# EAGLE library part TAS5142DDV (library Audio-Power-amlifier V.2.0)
STEREO DIGITAL AMPLIFIER POWER STAGE
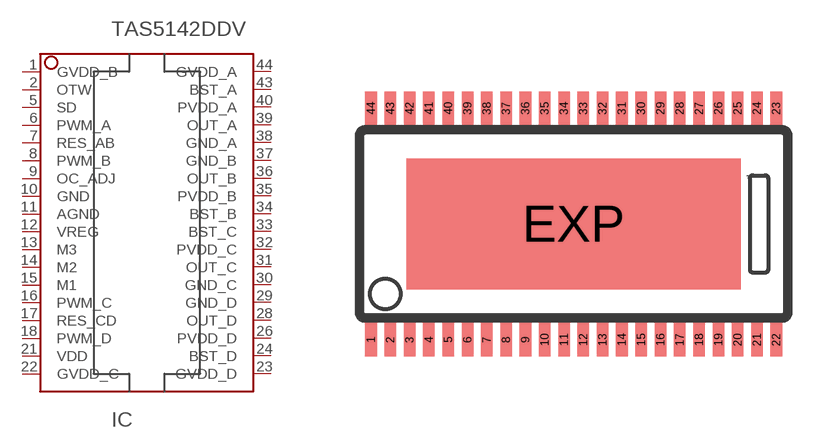
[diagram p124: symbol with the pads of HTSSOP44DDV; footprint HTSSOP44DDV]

Designator prefix IC

## TAS5142DDV  [HTSSOP44DDV]
1  GVDD_B
2  OTW  out
5  SD  out
6  PWM_A  in
7  RES_AB  in
8  PWM_B  in
9  OC_ADJ  out
10  GND  pwr
11  AGND  pwr
12  VREG  pwr
13  M3  in
14  M2  in
15  M1  in
16  PWM_C  in
17  RES_CD  in
18  PWM_D  in
21  VDD  pwr
22  GVDD_C  pwr
23  GVDD_D  pwr
24  BST_D  pwr
26  PVDD_D  pwr
28  OUT_D  out
29  GND_D  pwr
30  GND_C  pwr
31  OUT_C  out
32  PVDD_C  pwr
33  BST_C  pwr
34  BST_B  pwr
35  PVDD_B  pwr
36  OUT_B  out
37  GND_B  pwr
38  GND_A  pwr
39  OUT_A  out
40  PVDD_A  pwr
43  BST_A  pwr
44  GVDD_A  pwr

## Footprint HTSSOP44DDV (pad centres in mm)
PowerPAD(TM) PLASTIC SMALL-OUTLINE PACKAGE DDV (R-PDSO-G**) Source: http://focus.ti.com/lit/ml/mpds041b/mpds041b.pdf / slma002.pdf
smd 0.38 x 1.1: 1 -6.668,-3.81; 2 -6.032,-3.81; 3 -5.397,-3.81; 4 -4.763,-3.81; 5 -4.128,-3.81; 6 -3.493,-3.81; 7 -2.857,-3.81; 8 -2.223,-3.81; 9 -1.587,-3.81; 10 -0.953,-3.81; 11 -0.318,-3.81; 12 0.318,-3.81; 13 0.953,-3.81; 14 1.587,-3.81; 15 2.223,-3.81; 16 2.857,-3.81; 17 3.493,-3.81; 18 4.128,-3.81; 19 4.763,-3.81; 20 5.397,-3.81; 21 6.032,-3.81; 22 6.668,-3.81; 23 6.668,3.81; 24 6.032,3.81; 25 5.397,3.81; 26 4.763,3.81; 27 4.128,3.81; 28 3.493,3.81; 29 2.857,3.81; 30 2.223,3.81; 31 1.587,3.81; 32 0.953,3.81; 33 0.318,3.81; 34 -0.318,3.81; 35 -0.953,3.81; 36 -1.587,3.81; 37 -2.223,3.81; 38 -2.857,3.81; 39 -3.493,3.81; 40 -4.128,3.81; 41 -4.763,3.81; 42 -5.397,3.81; 43 -6.032,3.81; 44 -6.668,3.81
smd 11 x 4.3: EXP 0,0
